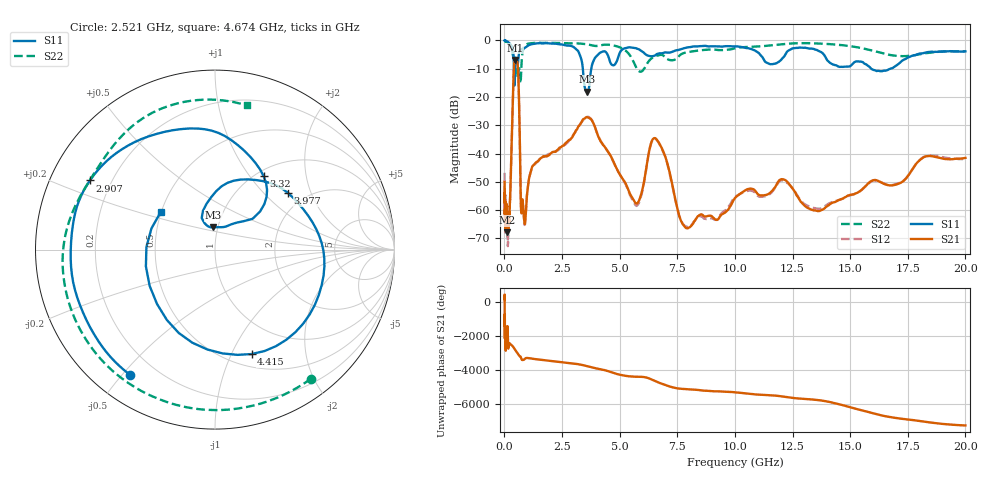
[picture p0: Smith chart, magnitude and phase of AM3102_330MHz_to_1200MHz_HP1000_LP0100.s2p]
! Date/Time: Tue, Sep 11, 2018 5:17 PM
! Network Analyzer: Agilent Technologies E8362B Rev: A.07.50.63
! Sweep from 0.010 to 20.000 GHz, 1601 Points, Sweep Type: LOG
! Power Supply: 4.949 V, 0.001 A
# Hz S DB R 50
!freq MagS11 AngS11 MagS21 AngS21 MagS12 AngS12 MagS22 AngS22
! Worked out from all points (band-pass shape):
!   1601 points, 10 MHz to 20 GHz, reference 50 ohm
!   highest |S21| = -6.91 dB at 458 MHz (marker M1); lowest = -67.9 dB at 123.4 MHz (marker M2)
!   |S21| within 3 dB of the highest: 412 MHz to 589.4 MHz (177.4 MHz wide, 35.4 % of centre)
!   lowest |S11| = -18.1 dB at 3.599 GHz (marker M3), VSWR 1.28, Z = 47.6 + j12 ohm
!   |S11| at or under -10 dB: 416.2 MHz to 466.5 MHz (50.32 MHz wide, 11.4 % of centre); 3.403 GHz to 3.77 GHz (366.3 MHz wide, 10.2 % of centre); 15.91 GHz to 16.76 GHz (841.6 MHz wide, 5.15 % of centre)
!   |S22| runs from -15.1 to -0.2 dB; largest |S21 - S12| = 0.0076
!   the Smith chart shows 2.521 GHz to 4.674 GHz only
!   S11 on the Smith chart (normalised r, x): 2.521 GHz: 0.11, -0.52; 2.907 GHz: 0.12, +0.25; 3.32 GHz: 1.09, +1.17; 3.977 GHz: 1.63, +1.40; 4.415 GHz: 0.64, -1.20; 4.674 GHz: 0.50, +0.24
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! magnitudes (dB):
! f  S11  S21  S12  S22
! 10 MHz  0.0  -50.0  -46.8  -0.2
! 35.55 MHz  0.0  -63.1  -65.0  -0.3
! 123.4 MHz  -0.4  -67.9  -63.4  -0.7
! 126.4 MHz  -0.4  -65.5  -64.2  -0.7
! 244.6 MHz  -1.2  -56.1  -56.6  -1.5
! 447.2 MHz  -15.4  -7.0  -7.1  -7.0
! 458 MHz  -12.5  -6.9  -7.0  -6.7
! 591.9 MHz  -7.7  -10.3  -10.4  -13.0
! 726 MHz  -3.2  -60.1  -60.3  -11.7
! 869.7 MHz  -2.7  -64.4  -65.1  -2.0
! 1.59 GHz  -1.0  -41.6  -41.5  -0.9
! 2.521 GHz  -1.5  -37.3  -37.5  -1.0
! 2.907 GHz  -2.0  -34.5  -34.3  -1.0
! 3.32 GHz  -6.2  -29.2  -29.2  -1.1
! 3.599 GHz  -18.1  -27.2  -27.0  -1.4
! 3.977 GHz  -5.8  -31.8  -31.7  -2.0
! 4.415 GHz  -4.2  -38.4  -38.3  -1.5
! 4.674 GHz  -8.7  -41.9  -42.0  -1.7
! 5.652 GHz  -2.6  -57.1  -57.8  -8.4
! 6.549 GHz  -5.2  -34.6  -34.8  -5.6
! 7.958 GHz  -2.5  -66.4  -65.9  -4.1
! 20 GHz  -3.9  -41.5  -42.1  -3.8
